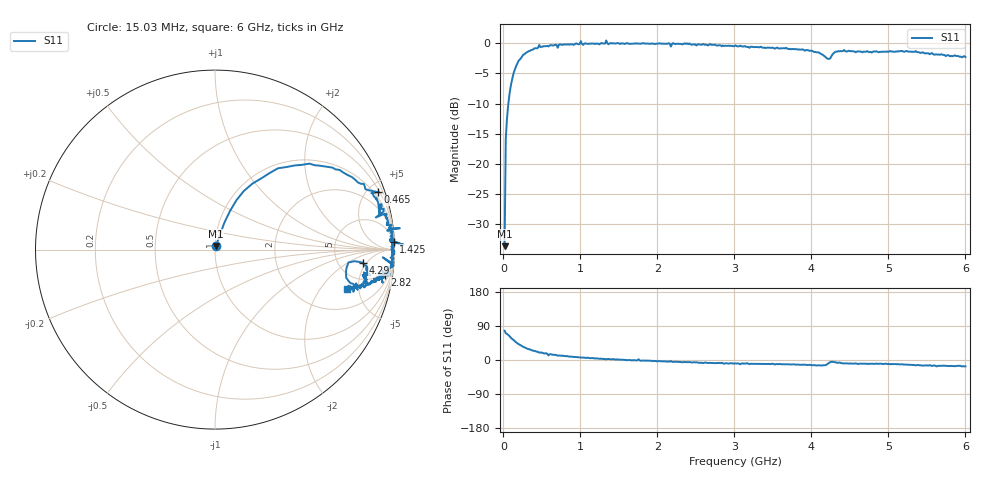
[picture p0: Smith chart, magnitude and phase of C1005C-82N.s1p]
!	Network	Analyzer	HP8753E.07.74:	Oct	30	2002	Serial	No.	JP38451487
!	Hewlett-Packard
!	28	Aug	2009	9:14:29
!	Frequency	S11
#	HZ	S	RI	R	50
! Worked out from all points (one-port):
!   400 points, 15.03 MHz to 6 GHz, reference 50 ohm
!   lowest |S11| = -33.6 dB at 15.03 MHz (marker M1), VSWR 1.04, Z = 50.4 + j2.06 ohm
!   |S11| at or under -10 dB: start of sweep to 63.98 MHz
!   S11 on the Smith chart (normalised r, x): 15.03 MHz: 1.01, +0.04; 465 MHz: 0.64, +5.78; 1.425 GHz: 3, +44; 2.82 GHz: 4, -12; 4.29 GHz: 8.66, -3.98; 6 GHz: 3.46, -3.69
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1.502992e7  0.00464 0.0204
3.002985e7  0.0526 0.151
6.00297e7  0.12 0.276
9.002955e7  0.209 0.368
1.350293e8  0.351 0.453
2.550287e8  0.654 0.457
4.650277e8  0.909 0.32
5.550272e8  0.897 0.289
5.850271e8  0.917 0.195
6.150269e8  0.928 0.253
7.650262e8  0.945 0.195
9.750251e8  0.968 0.119
1.005025e9  1.03 0.119
1.035025e9  0.959 0.106
1.320023e9  0.991 0.0462
1.335023e9  1.05 0.0271
1.365023e9  0.976 0.046
1.425023e9  0.996 0.0449
1.515022e9  0.982 0.0165
2.265019e9  0.983 -0.0817
2.820016e9  0.947 -0.14
3.015015e9  0.945 -0.154
3.765011e9  0.873 -0.174
4.200009e9  0.731 -0.157
4.290009e9  0.823 -0.0728
4.515007e9  0.848 -0.137
5.265004e9  0.83 -0.185
6e9  0.734 -0.22
